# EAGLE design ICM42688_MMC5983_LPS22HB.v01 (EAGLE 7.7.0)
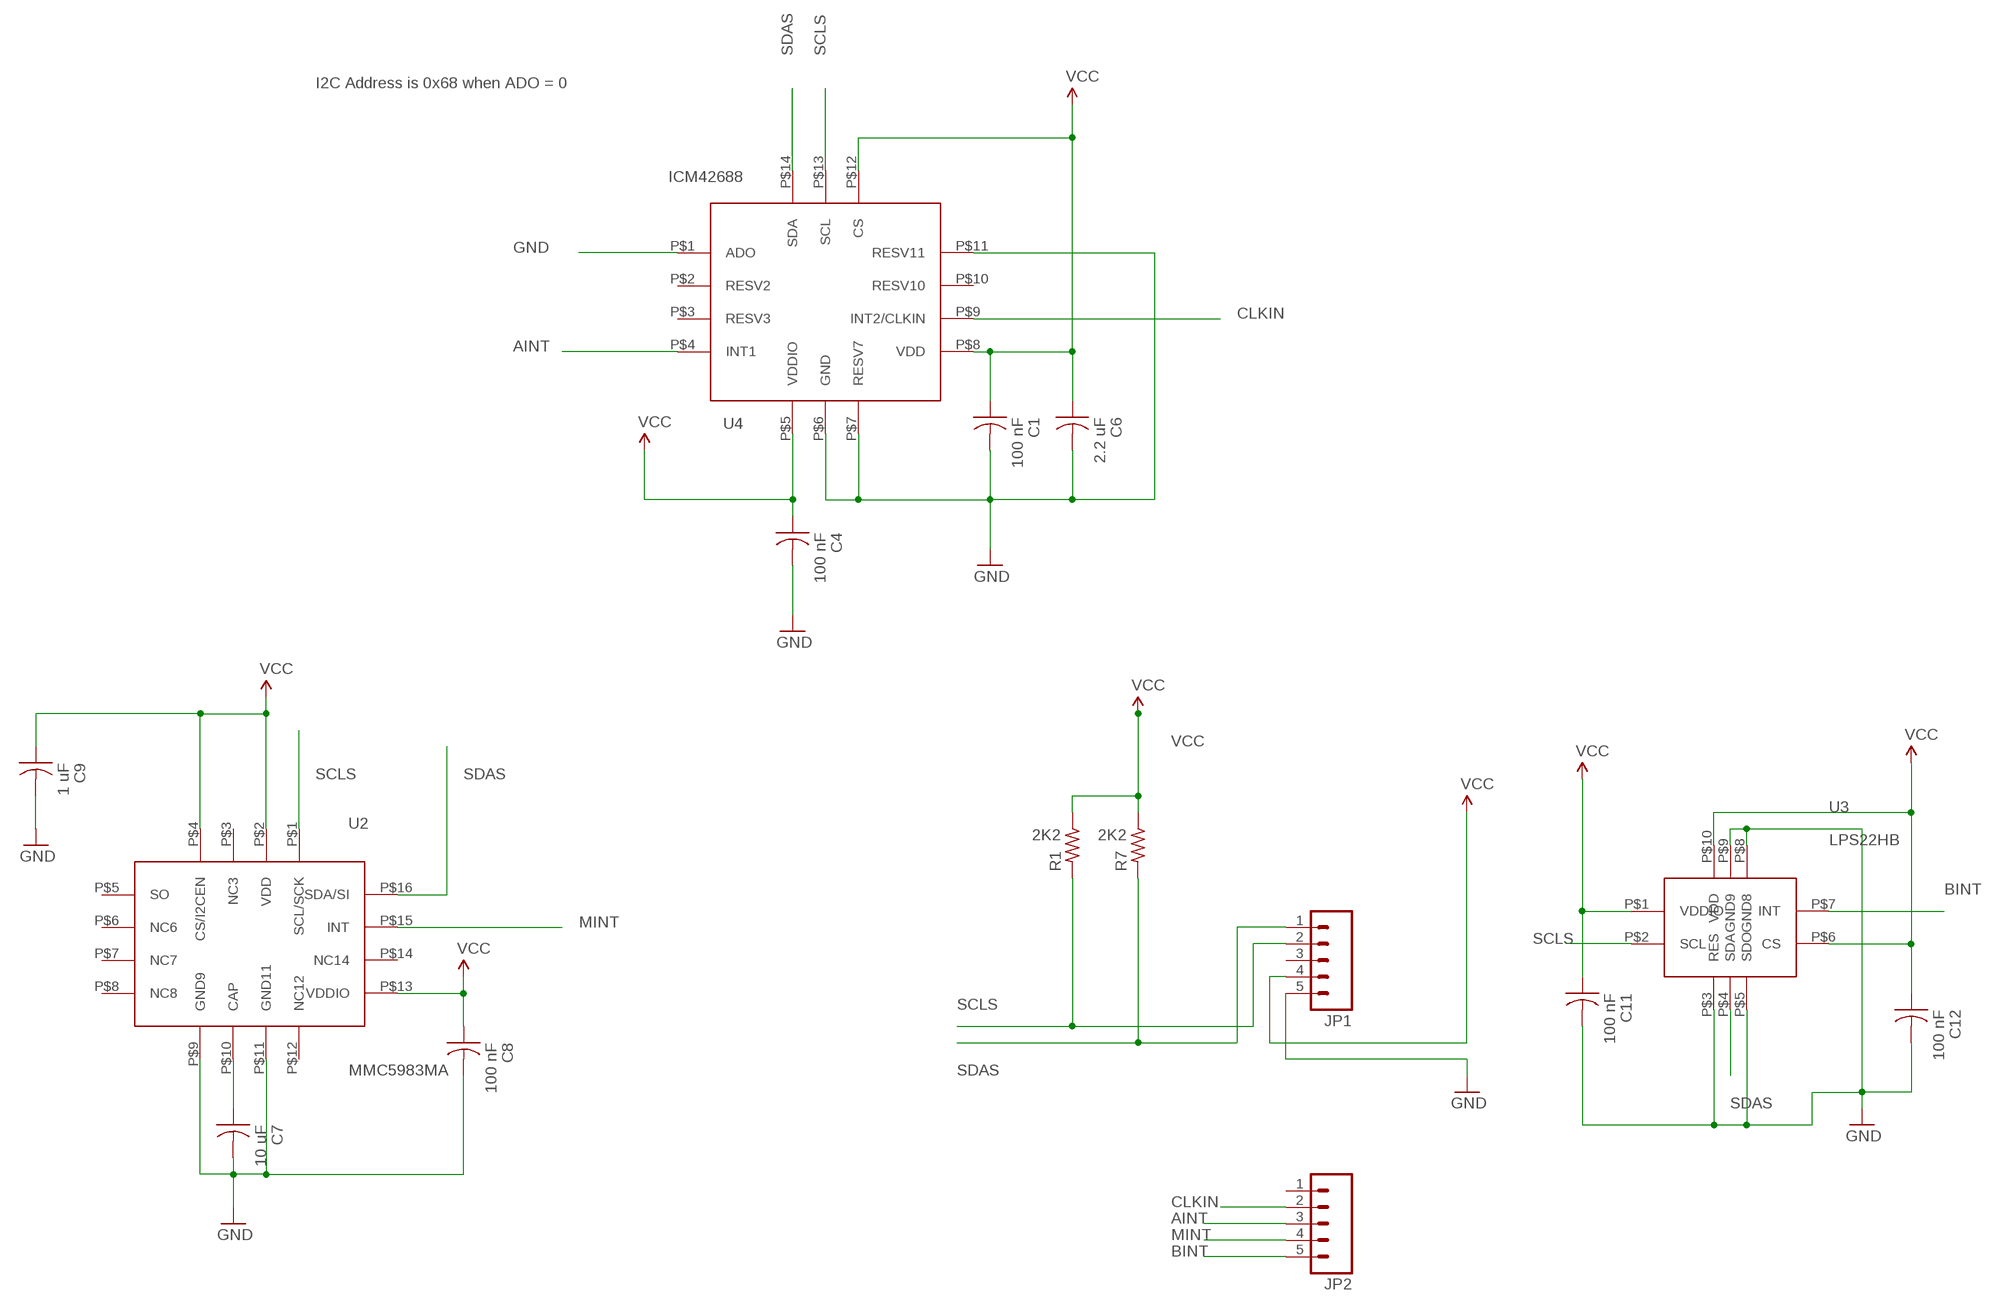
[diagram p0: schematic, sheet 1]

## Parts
C1  100 nF  C-US  [C0402_B]
C4  100 nF  C-US  [C0402_B]
C6  2.2 uF  C-US  [C0402_B]
C7  10 uF  C-US  [C0402_B]
C8  100 nF  C-US  [C0402_B]
C9  1 uF  C-US  [C0402_B]
C11  100 nF  C-US  [C0402_B]
C12  100 nF  C-US  [C0402_B]
JP1  M05NO_SILK  [1X05_NO_SILK]
JP2  M05NO_SILK  [1X05_NO_SILK]
R1  2K2  R-US_  [R0402_B]
R7  2K2  R-US_  [R0402_B]
U2  MMC5983MA  [MMC5983MA]
U3  LPS22HB  [LPS22HB]
U4  ICM42688  [ICM42688]

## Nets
AINT: JP2.3 U4.P$4(INT1)
BINT: JP2.5 U3.P$7(INT)
CLKIN: JP2.2 U4.P$9(INT2/CLKIN)
GND: C1.2 C4.2 C6.2 C7.2 C8.2 C9.2 C11.2 C12.2 JP1.5 U2.P$9(GND9) U2.P$11(GND11) U3.P$3(RES) U3.P$5(SDO) U3.P$8(GND8) U3.P$9(GND9) U4.P$1(ADO) U4.P$6(GND) U4.P$7(RESV7) U4.P$11(RESV11)
MINT: JP2.4 U2.P$15(INT)
N$2: C7.1 U2.P$10(CAP)
SCLS: JP1.2 R1.2 U2.P$1(SCL/SCK) U3.P$2(SCL) U4.P$13(SCL)
SDAS: JP1.1 R7.2 U2.P$16(SDA/SI) U3.P$4(SDA) U4.P$14(SDA)
VCC: C1.1 C4.1 C6.1 C8.1 C9.1 C11.1 C12.1 JP1.4 R1.1 R7.1 U2.P$2(VDD) U2.P$4(CS/I2CEN) U2.P$13(VDDIO) U3.P$1(VDDIO) U3.P$6(CS) U3.P$10(VDD) U4.P$5(VDDIO) U4.P$8(VDD) U4.P$12(CS)
Unconnected: JP1.3 JP2.1 U2.P$3(NC3) U2.P$5(SO) U2.P$6(NC6) U2.P$7(NC7) U2.P$8(NC8) U2.P$12(NC12) U2.P$14(NC14)

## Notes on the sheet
- I2C Address is 0x68 when ADO = 0

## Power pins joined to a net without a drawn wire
RESV2: U4.P$2(RESV2)
RESV3: U4.P$3(RESV3)
RESV10: U4.P$10(RESV10)

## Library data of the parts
C1 C4 C6-C9 C11 C12 = Spark:C-US: Capacitor
JP1 JP2 = SparkFun-Connectors:M05: Header 5 Standard 5-pin 0.1" header. Use with straight break away headers (SKU : PRT-00116), right angle break away headers (PRT-00553), swiss pins (PRT-00743), machine pins (PRT-00117), and female headers (PRT-00115). Molex polarized connector foot print use with SKU : PRT-08230 with associated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
R1 R7 = Spark:R-US_: 0402 Resistor
U2 = Kris:MMC5983MA: MMC5983MA ±8 Gauss, High Performance 3-axis Magnetic Sensor https://www.mouser.com/datasheet/2/821/Memsic_09102019_MMC5983MA_Datasheet_Rev_A-1635338.pdf
U3 = Kris:LPS22HB: LPS22HB ST pressure sensor http://www.st.com/content/ccc/resource/technical/document/datasheet/bf/c1/4f/23/61/17/44/8a/DM00140895.pdf/files/DM00140895.pdf/jcr:content/translations/en.DM00140895.pdf
U4 = Kris:ICM42688: TDK Invensense ICM42688 6-axis combo accel/gyro sensor https://3cfeqx1hf82y3xcoull08ihx-wpengine.netdna-ssl.com/wp-content/uploads/2021/06/DS-000347-ICM-42688-P-v1.5.pdf

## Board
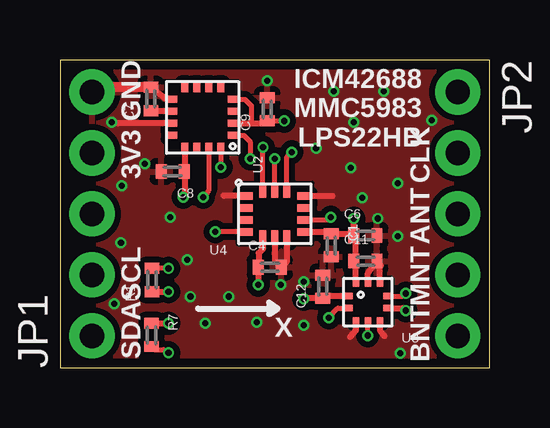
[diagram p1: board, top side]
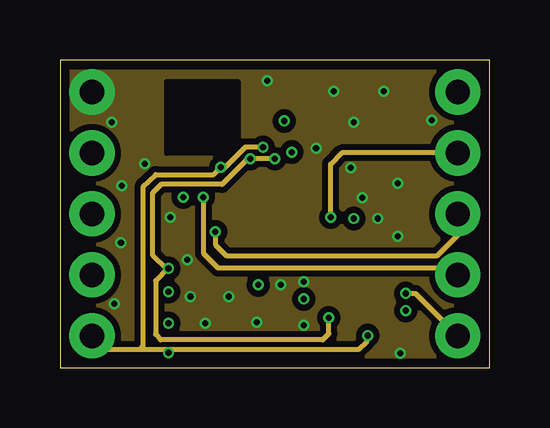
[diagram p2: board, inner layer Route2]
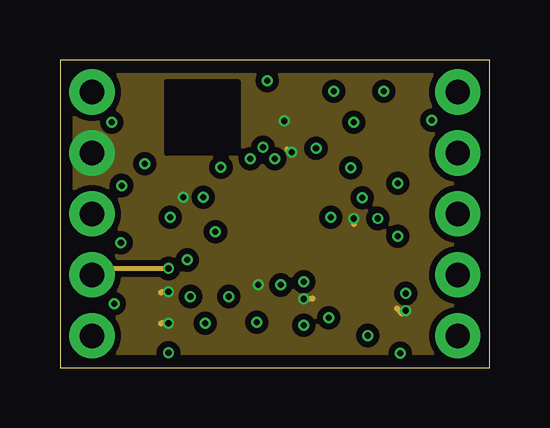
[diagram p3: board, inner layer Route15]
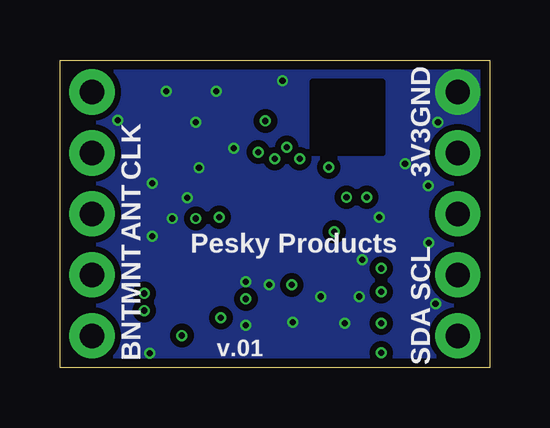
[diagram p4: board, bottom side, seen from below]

Size 17.91 x 12.83 mm. Coordinates in mm from the lower left corner, seen from the top.
Outline: 0,0 17.91,0 17.91,12.83 0,12.83 0,0
Copper layers (1*2*15*16): Top 0.035559375mm / dielectric 0.17018125mm / Route2 0.01778125mm / dielectric 47mil / Route15 0.01778125mm / dielectric 0.17018125mm / Bottom 0.035559375mm
Design rules "OSHPark-4layer *": minimum track width 5mil, minimum drill 10mil, track to track 5mil, track to pad 5mil, pad to pad 5mil, via to via 5mil, smd to smd 5mil, copper to edge 15mil, drill to drill 6mil, minimum pad ring 4mil, minimum via ring 4mil, stop-mask expansion 4mil, vias tented up to drill 20mil, thermal gap 10mil

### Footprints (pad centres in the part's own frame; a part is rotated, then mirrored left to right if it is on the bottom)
C0402_B = smd 0.457 x 0.61: 1 -0.483,0; 2 0.483,0
1X05_NO_SILK = drill 1.016 pad 1.88: 1 0,0; 2 2.54,0; 3 5.08,0; 4 7.62,0; 5 10.16,0
R0402_B = smd 0.457 x 0.61: 1 -0.483,0; 2 0.483,0
MMC5983MA = smd 0.3 x 0.45: P$1 0.75,1.275; P$2 0.25,1.275; P$3 -0.25,1.275; P$4 -0.75,1.275; P$9 -0.75,-1.275; P$10 -0.25,-1.275; P$11 0.25,-1.275; P$12 0.75,-1.275 | smd 0.45 x 0.3: P$5 -1.275,0.75; P$6 -1.275,0.25; P$7 -1.275,-0.25; P$8 -1.275,-0.75; P$13 1.275,-0.75; P$14 1.275,-0.25; P$15 1.275,0.25; P$16 1.275,0.75
LPS22HB = smd 0.3 x 0.275: P$1 -0.787,0.25; P$2 -0.787,-0.25; P$6 0.787,-0.25; P$7 0.787,0.25 | smd 0.275 x 0.3: P$3 -0.5,-0.787; P$4 0,-0.787; P$5 0.5,-0.787; P$8 0.5,0.787; P$9 0,0.787; P$10 -0.5,0.787
ICM42688 = smd 0.6 x 0.3: P$1 1.225,-0.75; P$2 1.225,-0.25; P$3 1.225,0.25; P$4 1.225,0.75; P$8 -1.225,0.75; P$9 -1.225,0.25; P$10 -1.225,-0.25; P$11 -1.225,-0.75 | smd 0.3 x 0.6: P$5 0.5,0.975; P$6 0,0.975; P$7 -0.5,0.975; P$12 -0.5,-0.975; P$13 0,-0.975; P$14 0.5,-0.975

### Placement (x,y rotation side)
C1  11.3,5.11 270 top
C4  8.74,4.19 0 top
C6  12.73,5.51 0 top
C7  3.78,11.2 90 top
C8  4.7,8.18 180 top
C9  8.64,10.77 90 top
C11  12.73,4.45 0 top
C12  10.95,3.38 90 top
JP1  1.33,1.33 90 top
JP2  16.57,11.49 270 top
R1  3.84,3.66 90 top
R7  3.81,1.37 270 top
U2  5.94,10.44 270 top
U3  12.83,2.74 0 top
U4  8.95,6.41 180 top

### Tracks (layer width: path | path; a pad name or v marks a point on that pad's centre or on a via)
AINT  (via drill 0.25)
  Top 0.203: U4.P$4 v6.48,5.66
  Route2 0.203: v6.48,5.66 6.48,5.13 6.93,4.67 15.72,4.67 16.57,5.52 JP2.3
BINT  (via drill 0.25)
  Top 0.203: U3.P$7 14.28,2.99 v14.4,3.1
  Route2 0.203: 16.45,1.33 JP2.5 14.81,3.1 v14.4,3.1
CLKIN  (via drill 0.25)
  Top 0.203: U4.P$9 11.17,6.16 v11.28,6.27
  Route2 0.203: v11.28,6.27 11.28,8.48 11.75,8.95 JP2.2
GND  (via drill 0.25)
  Top 0.203: 13.39,4.27 C11.2
  Top 0.254: U3.P$9 12.83,3.94 C11.2 13.33,4.17 U3.P$8 | U3.P$5 13.33,1.56 13.51,1.32 | U3.P$3 12.33,1.56 12.09,1.29 | U2.P$11 2.41,10.19 2.39,10.21 | U2.P$9 4.43,11.19 C7.2 | U4.P$11 11.35,7.16 | U4.P$6 8.95,4.46 C4.2 9.45,4.42 U4.P$7 | U4.P$1 6.83,7.16 6.81,7.19
  Top 0.406: C7.2 1.73,11.68 JP1.5
  other vias: 14.07,7.7 14.07,5.49 14.17,0.61 4.6,6.27 8.64,11.96 10.16,1.78 15.49,10.31 6.05,1.85 8.2,1.91 7.04,2.97 2.54,5.21 2.57,7.59 12.12,8.33 12.6,7.09 10.67,9.14 12.24,10.24 11.4,11.53 13.49,11.53 5.44,2.97 2.26,2.67 2.16,10.24 5.31,4.5 9.19,3.45 13.23,6.22 10.16,3.58 3.53,8.51
  pour Bottom (isolate 0.254, no thermals): 0,12.83 17.91,12.83 17.91,0 0,0
  pour Route2 (isolate 0.254, no thermals): 0,12.83 17.91,12.83 17.91,0 0,0
  pour Top (isolate 0.254): 0,12.83 17.91,12.83 17.91,0 0,0
MINT  (via drill 0.25)
  Top 0.203: U2.P$15 6.19,7.39 v5.97,7.11
  Route2 0.203: v5.97,7.11 5.97,4.78 6.58,4.17 16.28,4.17 JP2.4
N$1
  cutout Top: 4.45,11.94 7.42,11.94 7.42,8.94 4.45,8.94
  cutout Bottom: 4.45,11.94 7.42,11.94 7.42,8.94 4.45,8.94
  cutout Route2: 4.45,11.94 7.42,11.94 7.42,8.94 4.45,8.94
  cutout Route15: 4.45,11.94 7.42,11.94 7.42,8.94 4.45,8.94
N$2
  Top 0.254: U2.P$10 3.79,10.69 C7.1
N$3
  cutout Top: 11.84,3.73 13.82,3.73 13.82,1.78 11.84,1.78
N$5
  cutout Top: 7.42,7.7 10.49,7.7 10.49,5.16 7.42,5.16
SCLS  (via drill 0.25)
  Top 0.203: v11.2,2.08 11.58,2.49 U3.P$2 | U2.P$1 7.66,9.69 7.92,9.42 v7.92,8.71 | v4.52,4.14 R1.2 | U4.P$13 v8.95,8.71
  Route2 0.203: v8.95,8.71 v7.92,8.71 7.82,8.71 6.76,7.64 4.22,7.64 3.86,7.29 3.86,4.7 4.42,4.14 | v11.2,2.08 11.2,1.42 10.95,1.17 4.19,1.17 3.99,1.4 3.99,3.63 4.5,4.14 v4.52,4.14
  Route2 0.254: 4.42,4.14 v4.52,4.14
  Route15 0.203: JP1.2 1.69,3.87 1.96,4.14 v4.52,4.14
  Bottom 0.203: v11.2,2.08 11.18,1.96
SDAS  (via drill 0.25)
  Top 0.203: R7.2 3.94,0.76 4.32,0.76 v4.52,0.64 | v12.83,1.35 U3.P$4 | U2.P$16 6.69,8.42 v6.71,8.36 | U4.P$14 v8.45,9.19 v8.46,9.2
  Route2 0.203: 1.37,1.29 JP1.1 1.91,0.76 3.3,0.76 | 4.47,0.76 12.42,0.76 12.8,1.12 v12.83,1.35 | 4.47,0.76 3.3,0.76 | v8.46,9.2 7.72,9.2 6.77,8.24 6.71,8.31 v6.71,8.36 6.4,8.05 3.99,8.05 3.45,7.54 3.45,0.91 3.3,0.76 | v4.52,0.64 4.47,0.76
VCC  (via drill 0.25)
  Top 0.203: U2.P$4 7.71,11.19 7.98,10.92 7.98,10.21 7.95,10.19 | U4.P$12 9.45,8.79 v9.65,8.99 | C9.1 v9.35,10.29
  Top 0.254: U3.P$1 11.1,2.99 C12.1 10.19,2.9 v10.16,2.87 | 12.33,4.33 C11.1 12.33,4.36 | U3.P$6 14.27,2.49 v14.4,2.39 | R7.1 v4.52,1.85 | R1.1 v4.52,3.17 | U3.P$10 12.33,4.33 | 12.33,4.33 12.33,4.36 | U2.P$13 5.19,8.32 | 5.19,8.32 C8.1 | 5.19,8.32 5.19,7.15 v5.13,7.11 | U2.P$2 7.95,10.19 8.63,10.19 C9.1 | U4.P$8 11.23,5.66 C1.1 12.17,5.59 C6.1 | 12.33,4.36 12.33,5.43 C6.1 | C6.1 v12.24,6.22 12.24,6.33 | v8.26,3.45 C4.1 8.28,4.22 8.28,4.78 8.45,4.95 U4.P$5
  Route15 0.203: v9.65,8.99 9.45,9.12 9.47,9.09 | v9.35,10.29 9.27,10.19
  Route15 0.254: v10.16,2.87 10.52,2.9 | v12.24,6.22 12.24,5.99 | v14.4,2.39 14.25,2.26 14.05,2.46 | v4.52,1.85 4.22,1.85 | v4.52,3.17 4.22,3.15 | v5.13,7.11 5.13,7.16 5.16,7.19 | v8.26,3.45 8.26,3.53
  pour Route15 (isolate 0.254, no thermals): 0.64,12.19 17.27,12.19 17.27,0.64 10.54,0.64 10.52,0.64 0.64,0.64

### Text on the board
tPlace: ICM42688 / MMC5983 / LPS22HB | GND | CLK | 3V3 | ANT | MNT | SCL | BNT | X | SDA
bPlace: GND | 3V3 | CLK | ANT | Pesky Products | SCL | MNT | SDA | BNT | v.01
